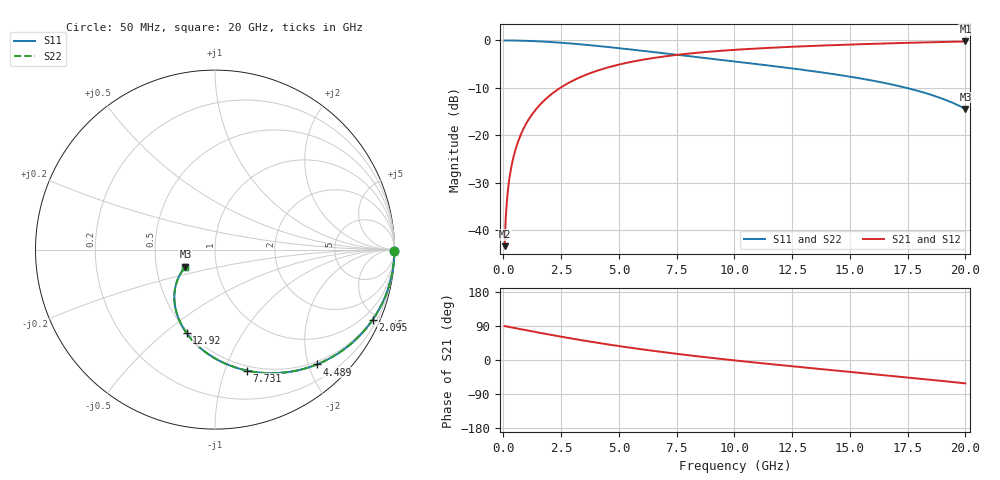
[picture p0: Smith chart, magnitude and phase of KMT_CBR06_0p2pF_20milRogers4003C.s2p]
! Data measured by Modelithics Inc. support@modelithics.com 813-866-6335
! KEMET CBR0603 0.2pF, Pad Width= 0.851mm, Pad Length= 0.64mm, Pad Gap= 0.62mm, 20mil Rogers 4003C substrate Data, January 2022
# hz S ma R 50
! 2 Port Network Data from SP1.SP block
! freq  magS11  angS11  magS21  angS21  magS12  angS12  magS22  angS22
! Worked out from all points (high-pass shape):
!   401 points, 50 MHz to 20 GHz, reference 50 ohm
!   highest |S21| = -0.22 dB at 20 GHz (marker M1); lowest = -43.3 dB at 50 MHz (marker M2)
!   |S21| within 3 dB of the highest: 7.2 GHz to end of sweep
!   lowest |S11| = -14.4 dB at 20 GHz (marker M3), VSWR 1.47, Z = 35.3 - j6.98 ohm
!   |S11| at or under -10 dB: 17.46 GHz to end of sweep
!   |S22| runs from -14.4 to 0.0 dB; largest |S21 - S12| = 0
!   S11 on the Smith chart (normalised r, x): 50 MHz: open; 2.095 GHz: 0.45, -4.66; 4.489 GHz: 0.45, -2.14; 7.731 GHz: 0.45, -1.19; 12.92 GHz: 0.49, -0.60; 20 GHz: 0.71, -0.14
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5e7  1 -0.6  0.006828 89.4  0.006828 89.4  1 -0.6
9.9875e7  0.9999 -1.2  0.01364 88.8  0.01364 88.8  0.9999 -1.2
1.99625e8  0.9996 -2.3  0.02725 87.7  0.02725 87.7  0.9996 -2.3
2.99375e8  0.9992 -3.5  0.04085 86.5  0.04085 86.5  0.9992 -3.5
4.49e8  0.9981 -5.3  0.06119 84.7  0.06119 84.7  0.9981 -5.3
5.98625e8  0.9966 -7.0  0.08145 83.0  0.08145 83.0  0.9966 -7.0
8.48e8  0.9933 -9.9  0.115 80.1  0.115 80.1  0.9933 -9.9
1.197125e9  0.9868 -13.9  0.1612 76.1  0.1612 76.1  0.9868 -13.9
1.596125e9  0.977 -18.5  0.2125 71.5  0.2125 71.5  0.977 -18.5
2.094875e9  0.9615 -24.0  0.2742 65.9  0.2742 65.9  0.9615 -24.0
3.391625e9  0.9083 -37.8  0.4172 52.2  0.4172 52.2  0.9083 -37.8
4.488875e9  0.855 -48.5  0.5171 41.4  0.5171 41.4  0.855 -48.5
5.53625e9  0.8023 -57.9  0.5952 32.0  0.5952 32.0  0.8023 -57.9
6.73325e9  0.7434 -67.7  0.6667 22.2  0.6667 22.2  0.7434 -67.7
7.73075e9  0.697 -75.2  0.7148 14.6  0.7148 14.6  0.697 -75.2
1.0025e10  0.6002 -90.9  0.7969 -1.2  0.7969 -1.2  0.6002 -90.9
1.291775e10  0.4921 -108.7  0.8669 -19.0  0.8669 -19.0  0.4921 -108.7
1.336662e10  0.4759 -111.3  0.8758 -21.7  0.8758 -21.7  0.4759 -111.3
1.506238e10  0.4134 -121.1  0.9063 -31.6  0.9063 -31.6  0.4134 -121.1
1.670825e10  0.3485 -130.6  0.9324 -41.3  0.9324 -41.3  0.3485 -130.6
1.850375e10  0.2684 -141.1  0.9576 -52.2  0.9576 -52.2  0.2684 -141.1
2e10  0.1903 -150.0  0.9752 -61.7  0.9752 -61.7  0.1903 -150.0
